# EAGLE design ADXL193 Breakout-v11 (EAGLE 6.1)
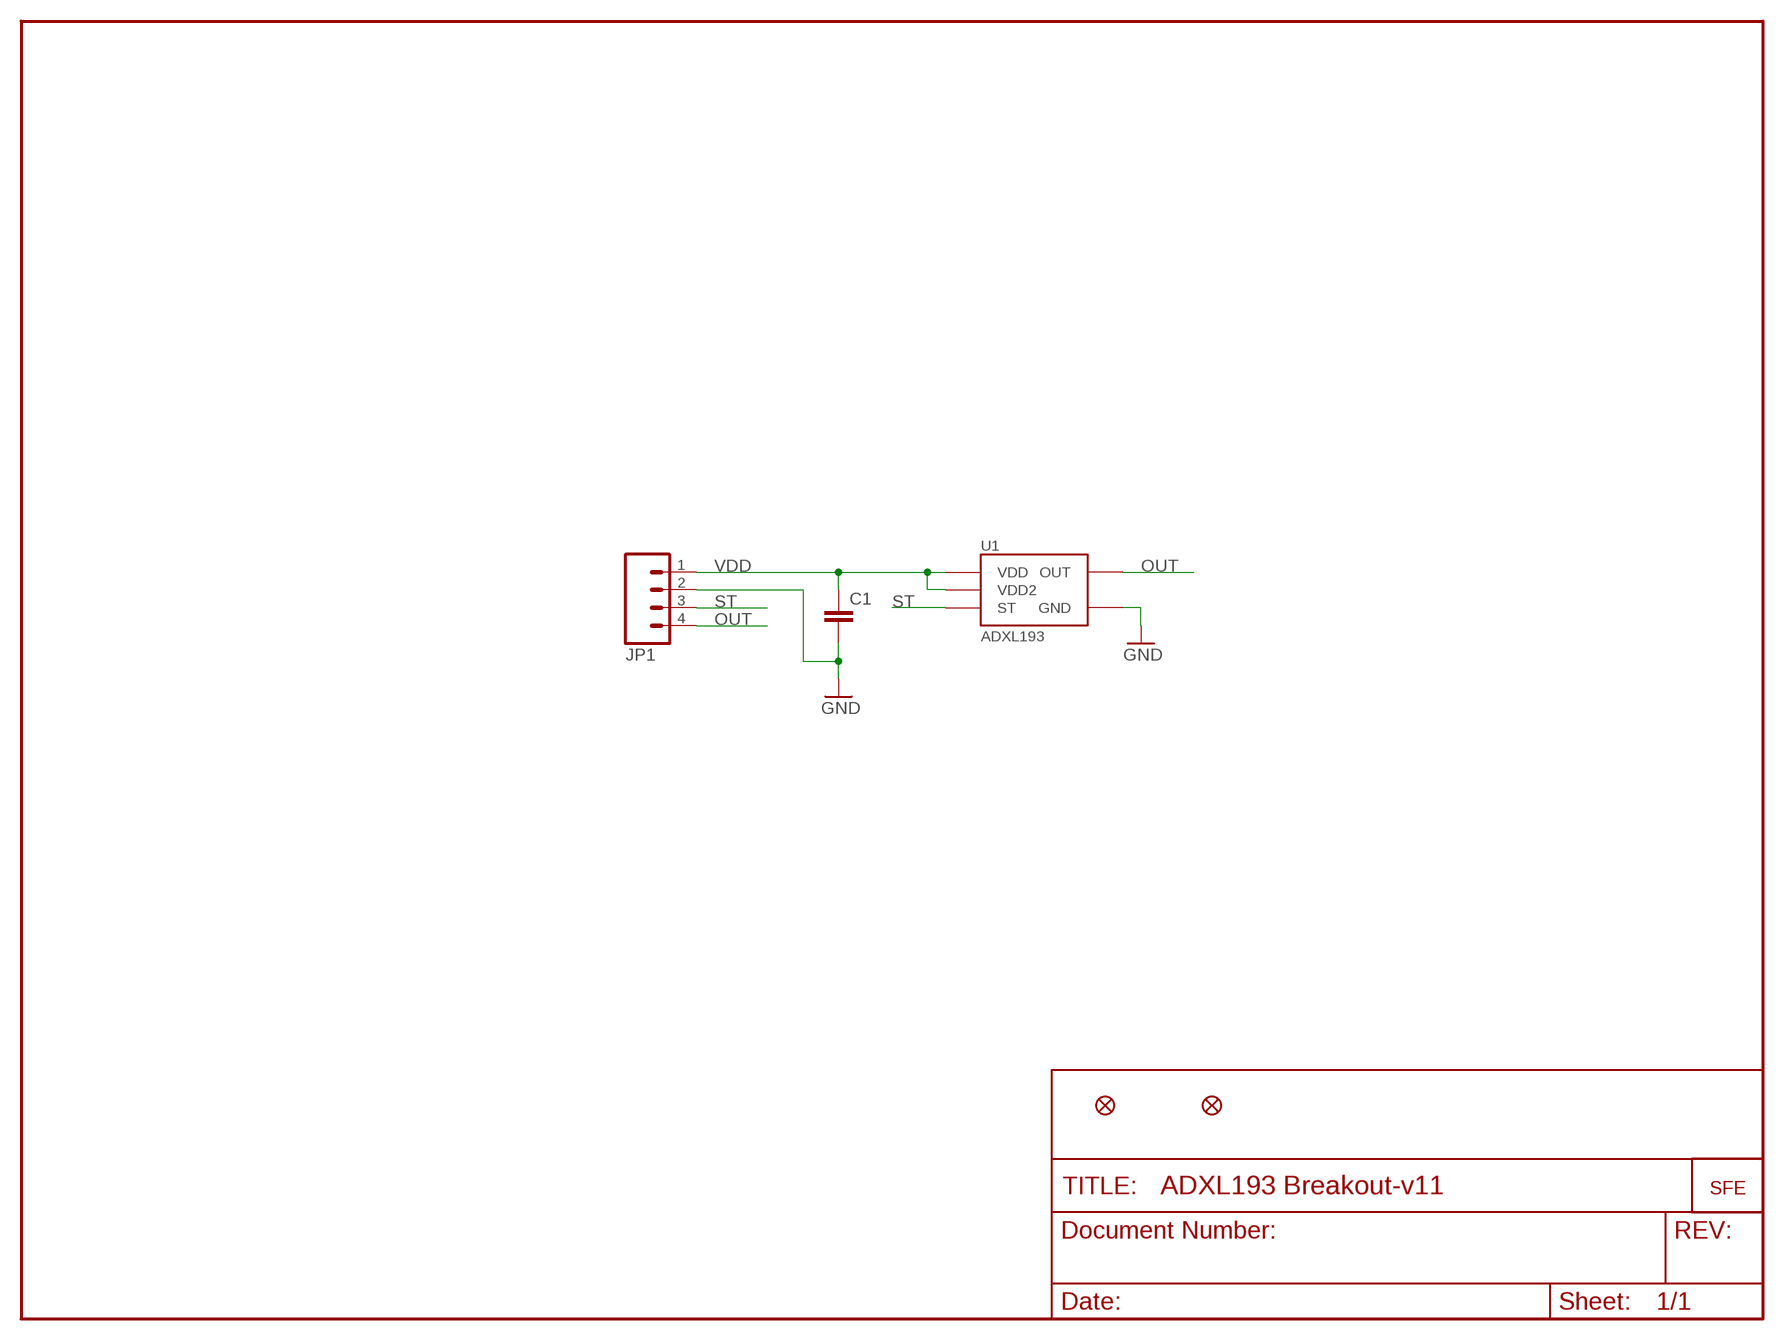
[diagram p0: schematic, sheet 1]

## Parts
C1  CAP0402-CAP  [0402-CAP]
JP1  M04PTH  [1X04]
JP2  FIDUCIALUFIDUCIAL  [MICRO-FIDUCIAL]
JP3  FIDUCIALUFIDUCIAL  [MICRO-FIDUCIAL]
U1  ADXL193  [ADXL193]
U$3  LOGO-SFESK  [SFE-LOGO-FLAME]

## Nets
GND: C1.2 JP1.2 U1.P$3(GND)
OUT: JP1.4 U1.P$6(OUT)
ST: JP1.3 U1.P$4(ST)
VDD: C1.1 JP1.1 U1.P$7(VDD) U1.P$8(VDD2)

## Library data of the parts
C1 = SparkFun:CAP: Capacitor
JP1 = SparkFun:M04: Header 4 Standard 4-pin 0.1" header. Use with straight break away headers (SKU : PRT-00116), right angle break away headers (PRT-00553), swiss pins (PRT-00743), machine pins (PRT-00117), and female headers (PRT-00115). Molex polarized connector foot print use with SKU : PRT-08231 with associated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
JP2 JP3 = SparkFun:FIDUCIAL: Fiducial Alignment Points
U1 = SparkFun:ADXL193: 250g accelerometer analog out
U$3 = SparkFun:LOGO-SFE: Spark Fun Electronics PCB Logo

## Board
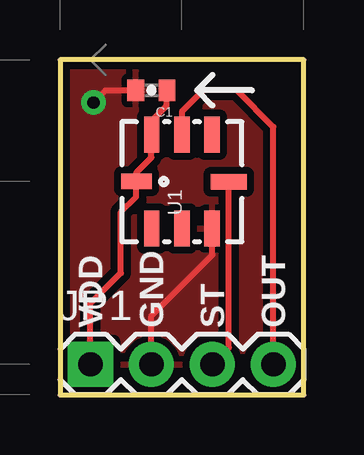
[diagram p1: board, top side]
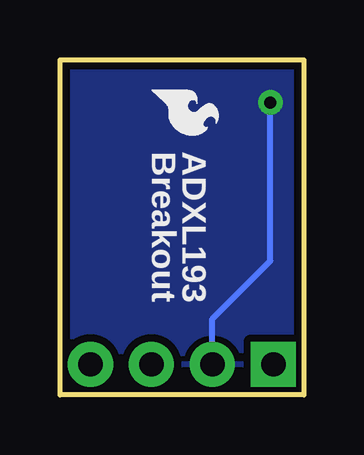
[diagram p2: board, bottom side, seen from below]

Size 10.16 x 13.97 mm. Coordinates in mm from the lower left corner, seen from the top.
Outline: 0,0 10.16,0 10.16,13.97 0,13.97 0,0
Copper layers (1*16): Top 0.035mm / dielectric 1.5mm / Bottom 0.035mm
Design rules: minimum track width 8mil, minimum drill 20mil, track to track 8mil, track to pad 8mil, pad to pad 8mil, via to via 8mil, smd to smd 8mil, copper to edge 9mil, drill to drill 8mil, minimum pad ring 12mil, minimum via ring 10mil, stop-mask expansion 4mil, vias tented up to drill 25mil, thermal gap 10mil

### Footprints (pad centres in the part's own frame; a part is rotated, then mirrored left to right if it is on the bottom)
0402-CAP = smd 0.7 x 0.9: 1 -0.65,0; 2 0.65,0
1X04 = drill 1.016 pad 1.88 square: 1 0,0 | drill 1.016 pad 1.88: 2 2.54,0; 3 5.08,0; 4 7.62,0
MICRO-FIDUCIAL = smd 0.635 x 0.635: 1 0,0
ADXL193 = smd 1.5 x 0.64: P$1 -1.96,1.26; P$2 -1.96,0; P$3 -1.96,-1.26; P$5 1.96,-1.26; P$6 1.96,0; P$7 1.96,1.26 | smd 0.64 x 1.5: P$4 0,-1.96 | smd 0.64 x 1.27: P$8 0.01,1.9

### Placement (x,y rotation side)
C1  3.81,12.7 180 top
JP1  1.27,1.27 0 top
JP2  not placed on the board
JP3  not placed on the board
U1  5.08,8.89 90 top
U$3  6.35,12.7 270 bottom

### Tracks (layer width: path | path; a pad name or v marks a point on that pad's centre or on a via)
GND  (via drill 0.51)
  Top 0.254: JP1.2 3.81,3.3 6.35,5.84 U1.P$3 | C1.2 1.91,12.7 v1.4,12.19
  Bottom 0.254: v1.4,12.19 1.4,5.59 3.81,3.17 JP1.2
  pour Top (isolate 0.305): 0,0 10.16,0 10.16,13.97 0,13.97
  pour Bottom (isolate 0.305): 0,0 10.16,0 10.16,13.97 0,13.97
OUT
  Top 0.254: U1.P$6 5.08,11.81 5.97,12.7 7.37,12.7 8.89,11.18 JP1.4
ST
  Top 0.254: U1.P$4 7.04,1.96 JP1.3
VDD
  Top 0.254: U1.P$8 | U1.P$8 3.18,9.28 3.81,9.91 U1.P$7 3.82,11.44 4.45,12.06 4.45,12.69 C1.1 | JP1.1 1.27,3.81 2.54,5.08 2.54,7.62 3.17,8.26 U1.P$8

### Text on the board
tPlace: VDD | GND | ST | OUT
bPlace: ADXL193 | Breakout
tDocu: 0.00" | 0.20" | 0.40" | 0.55" | 0.35" | 0.05" | 0.00"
